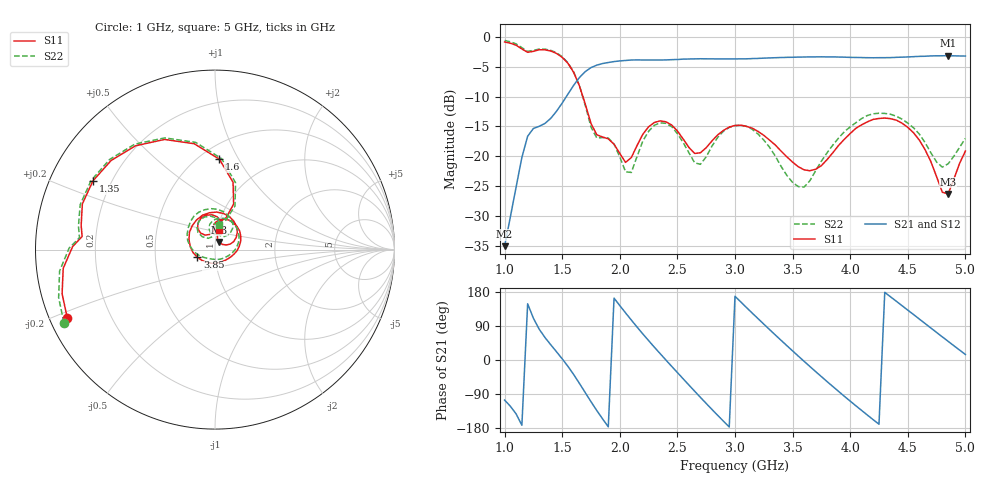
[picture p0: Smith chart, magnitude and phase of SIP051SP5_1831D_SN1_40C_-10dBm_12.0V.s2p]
# GHz  S  dB  R  50
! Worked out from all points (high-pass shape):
!   81 points, 1 GHz to 5 GHz, reference 50 ohm
!   highest |S21| = -3.14 dB at 4.85 GHz (marker M1); lowest = -35.1 dB at 1 GHz (marker M2)
!   |S21| within 3 dB of the highest: 1.683 GHz to end of sweep
!   lowest |S11| = -26.3 dB at 4.85 GHz (marker M3), VSWR 1.10, Z = 52.1 + j4.49 ohm
!   |S11| at or under -10 dB: 1.679 GHz to end of sweep
!   |S22| runs from -25.2 to -0.6 dB; largest |S21 - S12| = 0.0021
!   S11 on the Smith chart (normalised r, x): 1 GHz: 0.05, -0.22; 1.35 GHz: 0.13, +0.26; 1.6 GHz: 0.62, +0.84; 3.85 GHz: 0.82, -0.07; 5 GHz: 1.02, +0.22
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1  -0.84 -155.0  -35.05 -105.7  -34.88 -107.1  -0.59 -154.2
1.2  -2.57 174.4  -16.63 148.3  -16.61 148.3  -2.41 174.9
1.35  -2.15 150.6  -14.49 59.5  -14.50 59.5  -2.05 150.9
1.6  -5.95 87.2  -8.08 -38.6  -8.09 -38.6  -5.88 85.8
1.7  -11.24 67.7  -5.80 -86.1  -5.81 -86.2  -11.44 65.4
1.85  -16.76 90.8  -4.46 -155.2  -4.45 -155.3  -16.86 92.1
1.95  -17.97 91.3  -4.12 163.3  -4.14 163.3  -17.94 87.9
2.15  -18.18 131.1  -3.85 86.9  -3.85 86.9  -20.01 134.6
2.35  -14.07 104.2  -3.86 16.9  -3.86 16.8  -14.39 108.7
2.5  -15.75 79.0  -3.78 -33.1  -3.77 -33.1  -16.19 79.4
2.65  -19.52 81.2  -3.67 -82.4  -3.68 -82.5  -21.09 80.2
2.85  -16.40 89.0  -3.68 -146.1  -3.68 -146.1  -16.82 101.6
3  -14.83 65.6  -3.68 168.2  -3.68 168.1  -14.87 74.6
3.3  -17.29 8.2  -3.51 80.3  -3.51 80.4  -18.48 3.9
3.5  -20.97 -33.9  -3.40 24.0  -3.40 24.0  -24.38 -62.3
3.7  -22.17 -101.1  -3.34 -30.7  -3.33 -30.6  -22.41 -144.9
3.85  -19.38 -156.9  -3.34 -70.1  -3.35 -70.2  -18.09 -179.3
4.05  -15.29 145.9  -3.43 -121.0  -3.45 -121.0  -14.35 141.4
4.35  -13.69 77.2  -3.46 166.7  -3.46 166.7  -12.95 86.3
4.6  -17.28 30.1  -3.25 108.0  -3.25 108.1  -16.27 50.2
4.85  -26.30 62.6  -3.14 49.3  -3.15 49.3  -21.26 76.2
5  -19.12 77.6  -3.20 14.6  -3.21 14.7  -17.01 80.2
